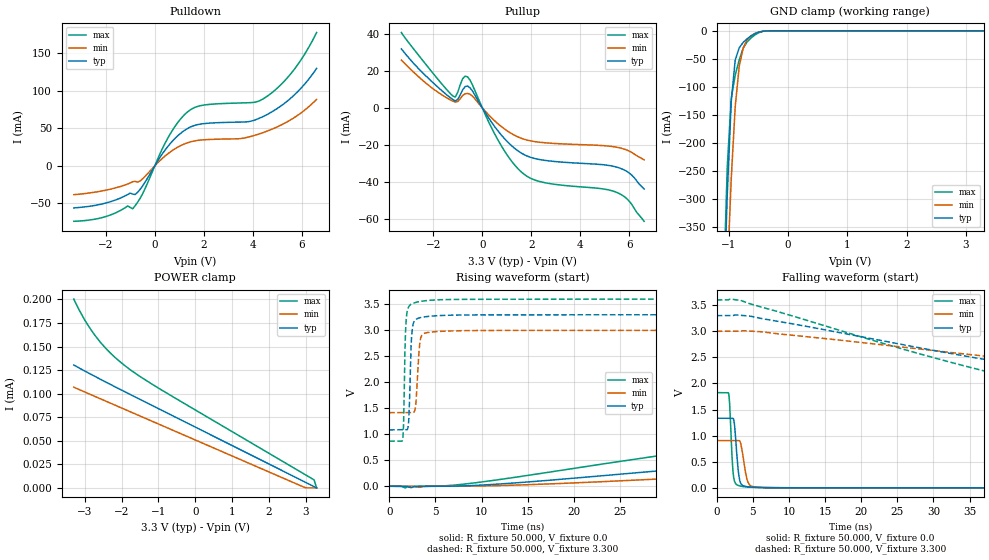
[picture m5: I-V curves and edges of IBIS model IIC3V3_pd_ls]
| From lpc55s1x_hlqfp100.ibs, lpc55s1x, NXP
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|   Model IIC3V3_pd_ls
[Model] IIC3V3_pd_ls
Model_type I/O
Polarity   Non-Inverting
Enable   Active-Low
Vinl =  0.990V
Vinh =  2.310V
Vmeas =  1.650V
Cref =  0.0F
Rref =  100.000
Vref =  0.0V
C_comp   2.367pF   2.322pF   2.392pF
C_comp_pullup   0.514pF   0.422pF   0.587pF
C_comp_pulldown   1.565pF   1.480pF   1.637pF
[Model Spec]
Vinh   2.310V   2.100V   2.520V
Vinl   0.990V   0.900V   1.080V
Vmeas   1.650V   1.500V   1.800V
Vref   0.0V   0.0V   0.0V
Cref   0.0F   0.0F   0.0F
Rref   100.000   100.000   100.000
[Temperature Range]   25.000   0.125k   -40.000
[Voltage Range]   3.300V   3.000V   3.600V
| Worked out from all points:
|   slope of the pulldown table from 0 to 0.495 V, typ, clamps not added: 20.4 ohm
|   slope of the pullup table from 0 to 0.495 V, typ, clamps not added: 49.8 ohm
|   GND clamp passes 1 mA (typ) near -0.43 V on its own axis
|   rising waveform, R_fixture 50.000, V_fixture 0.0: 20-80 % time 64.7ns typ, 78.1ns min, 51.2ns max; typ from 0 V to 1.32 V
|   rising waveform, R_fixture 50.000, V_fixture 3.300: 20-80 % time 237ps typ, 324ps min, 202ps max; typ from 1.08 V to 3.3 V
|   falling waveform, R_fixture 50.000, V_fixture 0.0: 20-80 % time 475ps typ, 657ps min, 378ps max; typ from 1.33 V to 0 V
|   falling waveform, R_fixture 50.000, V_fixture 3.300: 20-80 % time 50.7ns typ, 68.4ns min, 38.4ns max; typ from 3.3 V to 1.09 V
[Pulldown]
|Voltage   I(typ)   I(min)   I(max)
-3.3V     -56mA      -38.4mA    -73.87mA
-2.1V     -50.37mA   -33.07mA   -68.52mA
-1.1V     -38.15mA   -24.11mA   -53.37mA
-900mV    -37.61mA   -21.16mA   -57.18mA
-500mV    -26.92mA   -17.4mA    -37.43mA
500mV     24.51mA    15.34mA    35.14mA
1.2V      47.07mA    29.16mA    67.89mA
1.9V      55.94mA    34.55mA    80.54mA
3.8V      58.93mA    38.31mA    84.23mA
4.5V      67.15mA    45.39mA    91.04mA
5.6V      91.85mA    62.59mA    125mA
6.6V      130mA      88.72mA    177.8mA
[Pullup]
|Voltage   I(typ)   I(min)   I(max)
-3.3V     31.77mA    25.72mA    40.57mA
-2.2V     15.94mA    12.27mA    21.75mA
-1.2V     4.452mA    3.6mA      6.337mA
-1.1V     3.726mA    3.058mA    5.816mA
-800mV    9.696mA    6.594mA    15.7mA
-600mV    11.73mA    7.748mA    16.71mA
700mV     -13.46mA   -9.282mA   -18.76mA
1.7V      -25.21mA   -16.93mA   -35.78mA
2.6V      -28.44mA   -18.91mA   -40.52mA
5.5V      -32.06mA   -21.31mA   -45.71mA
6V        -35.26mA   -23.41mA   -50.46mA
6.6V      -43.76mA   -28.06mA   -61.21mA
[GND_clamp]
|Voltage   I(typ)   I(min)   I(max)
-3.3V     -10.05A    -9.18A     -11.33A
-1.089V   -516.5mA   -633.7mA   -475mA
-1.022V   -291.9mA   -436.3mA   -243.2mA
-955mV    -126mA     -264mA     -120.7mA
-888mV    -52.17mA   -135.6mA   -79.12mA
-821mV    -30.44mA   -63.69mA   -52.12mA
-754mV    -20.67mA   -30.69mA   -31.05mA
-687mV    -14.19mA   -15.97mA   -19.65mA
-553mV    -5.021mA   -4.512mA   -7.044mA
-419mV    -659.6uA   -714.3uA   -896.4uA
-285mV    -20.38uA   -37.42uA   -22.84uA
3.3V      0A         0A         0A
[POWER_clamp]
|Voltage   I(typ)   I(min)   I(max)
-3.3V     130.3uA    106.8uA    200.3uA
-3.132V   126.7uA    103.9uA    187.1uA
-2.998V   123.9uA    101.7uA    177.8uA
-2.73V    118.4uA    97.1uA     162.1uA
-2.529V   114.3uA    93.69uA    152.3uA
-2.328V   110.2uA    90.28uA    143.9uA
-1.926V   102.2uA    83.47uA    130.1uA
-1.524V   94.32uA    76.66uA    118.8uA
-921mV    82.52uA    66.44uA    104uA
2.965V    6.549uA    592.5nA    14.59uA
3.233V    1.309uA    0A         8.433uA
3.3V      0A         0A         0A
[Ramp]
| variable   typ   min   max
dV/dt_r   0.795/64.662n   0.534/78.103n   1.092/51.208n
dV/dt_f   1.328/50.650n   0.947/68.406n   1.639/38.349n
R_load = 50.000
[Rising Waveform]
R_fixture= 50.000
V_fixture= 0.0
V_fixture_min= 0.0
V_fixture_max= 0.0
|time   V(typ)   V(min)   V(max)
0s        10.23nV    71.93nV    30.73nV
1.74ns    77.63uV    89.5nV     -30.99mV
8.05ns    6.834mV    602.3uV    40.2mV
41.07ns   474.6mV    241.6mV    858.1mV
71.47ns   827.6mV    470.3mV    1.449V
84.41ns   980mV      550.4mV    1.616V
101.9ns   1.142V     652.5mV    1.725V
123.9ns   1.243V     768.4mV    1.782V
155.2ns   1.3V       849.3mV    1.81V
200ns     1.325V     889.4mV    1.821V
[Rising Waveform]
R_fixture= 50.000
V_fixture= 3.300
V_fixture_min= 3.000
V_fixture_max= 3.600
|time   V(typ)   V(min)   V(max)
0s        1.085V     1.415V     866.6mV
1.46ns    1.085V     1.415V     906.3mV
1.55ns    1.085V     1.415V     1.174V
1.76ns    1.085V     1.415V     2.955V
2ns       1.107V     1.415V     3.405V
2.57ns    3.107V     1.415V     3.519V
2.89ns    3.208V     1.606V     3.537V
3.37ns    3.243V     2.822V     3.555V
4.46ns    3.271V     2.964V     3.577V
200ns     3.298V     2.999V     3.598V
[Falling Waveform]
R_fixture= 50.000
V_fixture= 0.0
V_fixture_min= 0.0
V_fixture_max= 0.0
|time   V(typ)   V(min)   V(max)
0s        1.333V     906.1mV    1.824V
1.66ns    1.333V     906.1mV    1.805V
1.83ns    1.333V     906.1mV    1.514V
2.18ns    1.334V     906.1mV    454.3mV
2.46ns    1.207V     906.1mV    128.9mV
2.93ns    396mV      906.4mV    48.64mV
3.2ns     134.9mV    894.2mV    36.69mV
4.08ns    24.93mV    229.1mV    18.21mV
4.48ns    17.63mV    66.2mV     13.69mV
200ns     187.6nV    456.6nV    118.2nV
[Falling Waveform]
R_fixture= 50.000
V_fixture= 3.300
V_fixture_min= 3.000
V_fixture_max= 3.600
|time   V(typ)   V(min)   V(max)
0s        3.298V     2.999V     3.598V
3.37ns    3.304V     3.006V     3.588V
28.94ns   2.66V      2.645V     2.534V
49.04ns   2.193V     2.357V     1.837V
56.94ns   2.035V     2.258V     1.274V
66.03ns   1.791V     2.153V     1.025V
77.83ns   1.376V     2.026V     930.2mV
95.73ns   1.181V     1.723V     887.2mV
127.4ns   1.105V     1.489V     870.2mV
200ns     1.086V     1.421V     866.8mV
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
